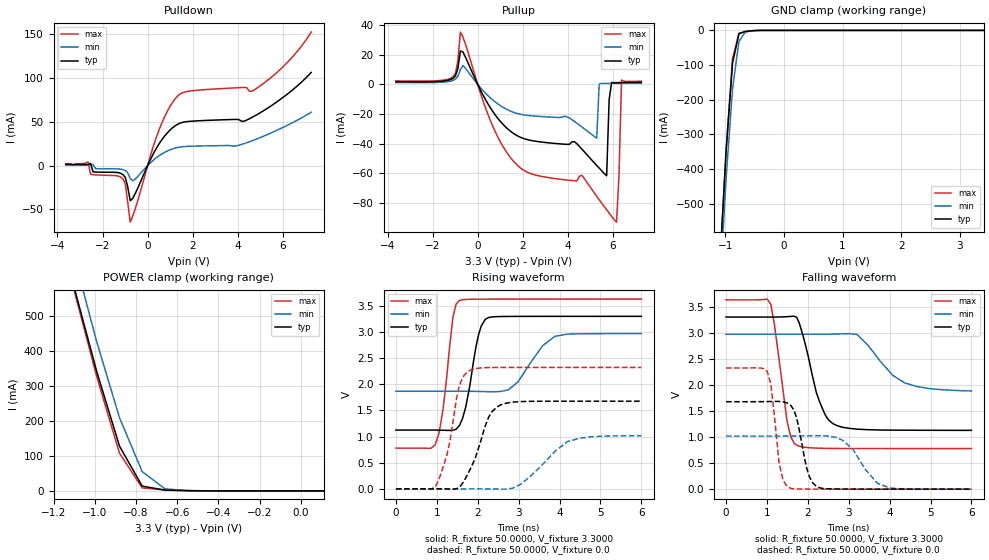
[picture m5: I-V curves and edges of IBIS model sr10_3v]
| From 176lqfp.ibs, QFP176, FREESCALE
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[Model] sr10_3v
|   Model sr10_3v
Model_type 3-state
Polarity   Non-Inverting
Enable   Active-High
Vmeas = 1.65
C_comp   4.7070pF   4.5257pF   4.9713pF
[Temperature Range]   25.0000   0.1500k   -40.0000
[Voltage Range]   3.3000V   2.9700V   3.6300V
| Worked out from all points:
|   slope of the pulldown table from 0 to 0.495 V, typ, clamps not added: 20.4 ohm
|   slope of the pullup table from 0 to 0.495 V, typ, clamps not added: 34.9 ohm
|   GND clamp passes 1 mA (typ) near -0.56 V on its own axis
|   POWER clamp passes 1 mA (typ) near -0.57 V on its own axis
|   rising waveform, R_fixture 50.0000, V_fixture 3.3000: 20-80 % time 293ps typ, 584ps min, 247ps max; typ from 1.12 V to 3.3 V
|   rising waveform, R_fixture 50.0000, V_fixture 0.0: 20-80 % time 463ps typ, 815ps min, 344ps max; typ from 0 V to 1.68 V
|   falling waveform, R_fixture 50.0000, V_fixture 3.3000: 20-80 % time 440ps typ, 765ps min, 285ps max; typ from 3.3 V to 1.13 V
|   falling waveform, R_fixture 50.0000, V_fixture 0.0: 20-80 % time 268ps typ, 572ps min, 190ps max; typ from 1.68 V to 0 V
[Pulldown]
|Voltage   I(typ)   I(min)   I(max)
-3.63V    1.32mA     750uA      2.18mA
-2.64V    1.318mA    673uA      4.109mA
-2.53V    2.439mA    685uA      -9.768mA
-2.42V    -7.096mA   1.248mA    -10.39mA
-1.1V     -10.06mA   -4.495mA   -14.98mA
-990mV    -13.52mA   -5.552mA   -20.79mA
-770mV    -40.02mA   -14.62mA   -64.52mA
440mV     22mA       9.997mA    36.03mA
1.32V     46.99mA    20.63mA    79.09mA
4.62V     54.83mA    28.22mA    84.86mA
6.16V     80.76mA    45.47mA    116.6mA
7.26V     106.3mA    60.95mA    152.3mA
[Pullup]
|Voltage   I(typ)   I(min)   I(max)
-3.63V    1.83mA     1.29mA     2.38mA
-1.1V     4.083mA    2.698mA    5.131mA
-770mV    22.7mA     10.09mA    35.47mA
1.54V     -32.68mA   -18.57mA   -51.17mA
5.28V     -54.85mA   -36.38mA   -75.78mA
5.39V     -56.66mA   304uA      -78.12mA
5.72V     -61.84mA   686uA      -84.88mA
5.83V     -10.4mA    697uA      -87.12mA
6.16V     1.209mA    726uA      -93.29mA
6.27V     1.231mA    734uA      -60.72mA
6.38V     1.249mA    742uA      2.96mA
7.26V     1.36mA     800uA      2.18mA
[GND_clamp]
|Voltage   I(typ)   I(min)   I(max)
-3.63V    -10.3A     -10.22A    -10.42A
-1.1V     -683.5mA   -753.4mA   -695.2mA
-990mV    -349.5mA   -429.8mA   -348.6mA
-880mV    -94.6mA    -168.5mA   -81.77mA
-770mV    -9.279mA   -31.37mA   -8.241mA
-660mV    -2.916mA   -4.583mA   -4.405mA
-440mV    -65.66uA   -239.8uA   -36.5uA
3.41V     626.5pA    220.2uA    6.002pA
[POWER_clamp]
|Voltage   I(typ)   I(min)   I(max)
-3.63V    7.308A     7.439A     7.307A
-1.1V     583.2mA    670.8mA    574.6mA
-990mV    341mA      426.7mA    326.9mA
-880mV    128.5mA    209.9mA    108.2mA
-770mV    13.88mA    55.46mA    8.675mA
-660mV    2.265mA    6.121mA    3.037mA
-550mV    681.9uA    981.3uA    900.8uA
110mV     37.89pA    5.502nA    6.134pA
[Ramp]
| variable   typ   min   max
dV/dt_r  1.0061/0.4627n   0.6102/0.7734n   1.3939/0.3398n
dV/dt_f  1.3036/0.4403n   0.6524/0.7314n   1.7106/0.2815n
R_load = 50.0000
[Rising Waveform]
R_fixture= 50.0000
V_fixture= 3.3000
V_fixture_min= 2.9700
V_fixture_max= 3.6300
|time   V(typ)   V(min)   V(max)
0s        1.125V     1.867V     778.9mV
959.4ps   1.125V     1.867V     840.4mV
1.153ns   1.121V     1.867V     1.526V
1.394ns   1.122V     1.867V     3.285V
1.554ns   1.212V     1.867V     3.604V
2.024ns   2.958V     1.863V     3.628V
2.182ns   3.241V     1.86V      3.629V
2.754ns   3.298V     1.897V     3.629V
3.887ns   3.299V     2.917V     3.63V
6ns       3.3V       2.969V     3.63V
[Rising Waveform]
R_fixture= 50.0000
V_fixture= 0.0
V_fixture_min= 0.0
V_fixture_max= 0.0
|time   V(typ)   V(min)   V(max)
0s        101.7nV    183.9nV    329.2nV
964.9ps   448.9uV    40.01uV    39.37mV
1.243ns   -737.7uV   17.76uV    641.3mV
1.534ns   23.92mV    37.14uV    1.92V
1.844ns   421.7mV    373.5uV    2.279V
2.268ns   1.374V     -142.4uV   2.32V
2.566ns   1.607V     -3.77mV    2.322V
3.049ns   1.669V     86.56mV    2.323V
4.198ns   1.677V     904.8mV    2.323V
6ns       1.677V     1.017V     2.323V
[Falling Waveform]
R_fixture= 50.0000
V_fixture= 3.3000
V_fixture_min= 2.9700
V_fixture_max= 3.6300
|time   V(typ)   V(min)   V(max)
0s        3.3V       2.97V      3.63V
1.096ns   3.3V       2.97V      3.541V
1.488ns   3.306V     2.97V      1.323V
1.58ns    3.312V     2.97V      1.008V
1.729ns   3.292V     2.97V      843mV
2.205ns   1.86V      2.97V      787.2mV
2.62ns    1.253V     2.973V     781mV
3.204ns   1.151V     2.965V     779.3mV
4.377ns   1.13V      2.034V     779mV
6ns       1.127V     1.883V     779mV
[Falling Waveform]
R_fixture= 50.0000
V_fixture= 0.0
V_fixture_min= 0.0
V_fixture_max= 0.0
|time   V(typ)   V(min)   V(max)
0s        1.677V     1.018V     2.323V
1.007ns   1.679V     1.018V     2.26V
1.097ns   1.681V     1.018V     2.004V
1.295ns   1.682V     1.018V     509.8mV
1.492ns   1.654V     1.018V     49.57mV
1.718ns   1.383V     1.02V      4.029mV
2.207ns   53.88mV    1.025V     667.9uV
2.851ns   2.522mV    938mV      160.7uV
4.005ns   715.3uV    21.53mV    56.49uV
6ns       273.7uV    763.6uV    10.34uV
